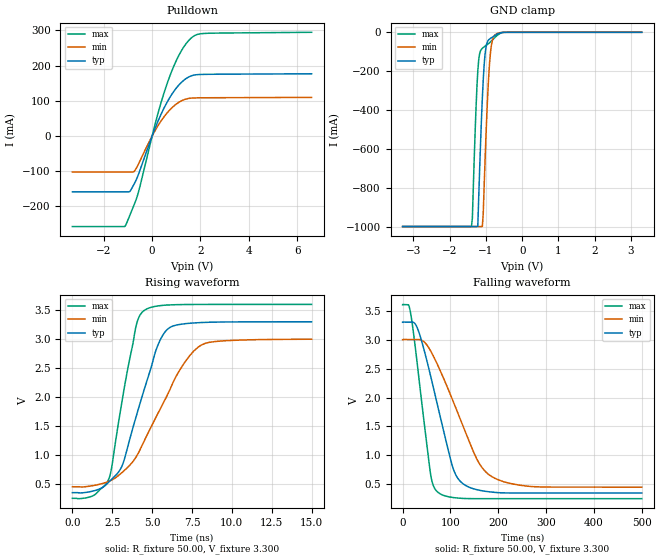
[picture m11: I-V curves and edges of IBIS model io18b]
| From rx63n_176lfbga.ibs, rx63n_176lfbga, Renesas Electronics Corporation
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[Model]   io18b
Model_type   I/O_open_drain
Polarity   Non-Inverting
Enable   Active-High
Vinl  =   0.990V
Vinh  =   2.310V
Vmeas =   1.650V
Rref  =   882.000
Cref  =   30.00pF
Vref  =   3.300V
| variable   typ   min   max
C_comp   8.300pF   8.300pF   8.300pF
| variable   typ   min   max
[Temperature Range]   45.000   105.000   -40.000
| variable   typ   min   max
[Voltage Range]   3.300V   3.000V   3.600V
| variable   typ   min   max
[Pulldown Reference]   0.000V   0.000V   0.000V
| variable   typ   min   max
[POWER Clamp Reference] 3.300V   3.000V   3.600V
| variable   typ   min   max
[GND Clamp Reference]   0.000V   0.000V   0.000V
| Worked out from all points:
|   slope of the pulldown table from 0 to 0.495 V, typ, clamps not added: 6.19 ohm
|   GND clamp passes 1 mA (typ) near -0.55 V on its own axis
|   rising waveform, R_fixture 50.00, V_fixture 3.300: 20-80 % time 1.86ns typ, 2.8ns min, 1.26ns max; typ from 0.35 V to 3.3 V
|   falling waveform, R_fixture 50.00, V_fixture 3.300: 20-80 % time 51.5ns typ, 76.6ns min, 29ns max; typ from 3.3 V to 0.35 V
[Pulldown]
| io18b_strong Pulldown rx631_rx63n
| Thu Mar 22 17:15:49 2012
| voltage   I(typ)   I(min)   I(max)
-3.3V     -158.4mA   -102mA     -257mA
-1.125V   -158.4mA   -102mA     -256.5mA
-925mV    -157.4mA   -102mA     -225.3mA
-725mV    -133.5mA   -98.66mA   -191.7mA
-525mV    -101.1mA   -73.63mA   -148.5mA
200mV     35.26mA    24.64mA    53.81mA
650mV     99.95mA    68.22mA    154.9mA
1.15V     148.2mA    97.72mA    234.9mA
1.4V      163.1mA    105.1mA    262mA
1.65V     171.7mA    108mA      280.4mA
2.2V      175.3mA    108.8mA    291.7mA
6.6V      177mA      109.9mA    294.8mA
[GND Clamp]
| io18b_strong GNDClamp rx631_rx63n
| Thu Mar 22 17:15:49 2012
| voltage   I(typ)   I(min)   I(max)
-3.3V     -1A        -1A        -1A
-1.4V     -1A        -1A        -1A
-1.375V   -1A        -1A        -957.7mA
-1.3V     -1A        -1A        -520.4mA
-1.225V   -998.5mA   -1A        -199.4mA
-1.1V     -340.9mA   -1A        -82.54mA
-1.075V   -245mA     -934.1mA   -78.46mA
-1.025V   -113.1mA   -661.3mA   -71.17mA
-900mV    -34.58mA   -157.8mA   -53.45mA
-800mV    -21.93mA   -28.23mA   -35.44mA
-625mV    -4.233mA   -2.444mA   -7.524mA
3.3V      0A         0A         0A
[POWER Clamp]
| io18b_strong PWRClamp rx631_rx63n
| Thu Mar 22 17:15:49 2012
| voltage   I(typ)   I(min)   I(max)
-3.3V     0A         0A         0A
0V        0A         0A         0A
3.3V      0A         0A         0A
[Ramp]
dV/dt_r   1.770/1.86n   1.529/2.80n   2.009/1.26n
dV/dt_f   1.770/51.51n   1.529/76.49n   2.009/29.00n
R_load = 50.00ohm
[Rising Waveform]
| io18b_strong Rising-High rx631_rx63n
| Thu Mar 22 17:15:49 2012
R_fixture = 50.00
V_fixture = 3.300
V_fixture_min = 3.000
V_fixture_max = 3.600
C_fixture = 0.00pF
| Time   V(typ)   V(min)   V(max)
0s        350mV      451mV      252mV
1.325ns   380mV      473mV      301mV
2.295ns   536mV      546mV      594mV
3.12ns    816mV      700mV      1.943V
3.955ns   1.624V     949mV      3.18V
4.46ns    2.093V     1.218V     3.487V
5.275ns   2.835V     1.67V      3.57V
5.835ns   3.134V     1.97V      3.587V
8.02ns    3.286V     2.887V     3.599V
15ns      3.3V       2.999V     3.6V
[Falling Waveform]
| io18b_strong Falling-High rx631_rx63n
| Thu Mar 22 17:15:49 2012
R_fixture = 50.00
V_fixture = 3.300
V_fixture_min = 3.000
V_fixture_max = 3.600
C_fixture = 0.00pF
| Time   V(typ)   V(min)   V(max)
0s        3.3V       3V         3.6V
16.04ns   3.303V     3.002V     3.49V
31.99ns   3.177V     3.002V     2.487V
58.45ns   2.376V     2.807V     680mV
73.98ns   1.832V     2.55V      361mV
114.5ns   615mV      1.752V     264mV
156.6ns   405mV      914mV      252mV
186.6ns   366mV      633mV      252mV
270.5ns   350mV      461mV      252mV
500ns     350mV      451mV      252mV
